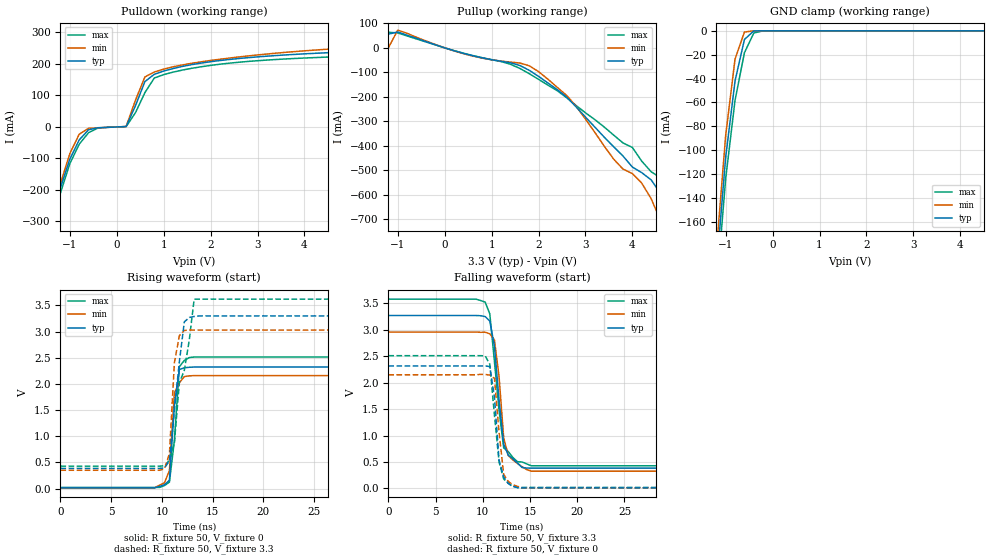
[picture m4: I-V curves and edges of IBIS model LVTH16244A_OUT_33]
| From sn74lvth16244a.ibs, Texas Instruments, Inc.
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|  Model LVTH16244A OUTPUT_33
[Model]   LVTH16244A_OUT_33
Model_type  3-state
Polarity   Inverting
Enable   Active-Low
Vmeas = 1.5V
Cref = 50pF
Rref = 500
Vref = 0
| variable   typ   min   max
C_comp   9pf   NA   NA
[Temperature Range]   40   -25   100
| Ambient temperature   25   -40   85
[Voltage range]   3.3   3.0   3.6
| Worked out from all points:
|   slope of the pulldown table from 0 to 0.495 V, typ, clamps not added: 4.75 ohm
|   slope of the pullup table from 0 to 0.495 V, typ, clamps not added: 18.1 ohm
|   GND clamp passes 1 mA (typ) near -0.43 V on its own axis
|   rising waveform, R_fixture 50, V_fixture 0: 20-80 % time 578ps typ, 424ps min, 626ps max; typ from 0.013 V to 2.32 V
|   falling waveform, R_fixture 50, V_fixture 3.3: 20-80 % time 906ps typ, 867ps min, 1.08ns max; typ from 3.27 V to 0.384 V
|   rising waveform, R_fixture 50, V_fixture 3.3: 20-80 % time 946ps typ, 513ps min, 1.47ns max; typ from 0.386 V to 3.3 V
|   falling waveform, R_fixture 50, V_fixture 0: 20-80 % time 696ps typ, 699ps min, 798ps max; typ from 2.32 V to 0.01 V
[Pullup]
|  Voltage   I(typ)   I(min)   I(max)
-5V       75.18uA    69.08uA    78.73uA
-2V       66.13uA    58.35uA    71.21uA
-1.8V     54.42mA    58.13uA    70.93uA
-1.6V     54.34mA    57.93uA    70.68uA
-1.2V     55.85mA    57.48uA    63.46mA
-1V       64.85mA    72.21mA    61.01mA
2V        -116.5mA   -96.95mA   -128.6mA
4.2V      -509.9mA   -552.6mA   -463mA
4.6V      -594.6mA   -704.6mA   -530.6mA
5V        -741.4mA   -898.7mA   -629.6mA
5.4V      -902.7mA   -1.093A    -764.1mA
10V       -2.757A    -3.325A    -2.409A
[Pulldown]
|   Voltage   I(typ)   I(min)   I(max)
-5V       -2.912A    -3.255A    -2.64A
-1.4V     -305mA     -304mA     -322.6mA
-1V       -102.1mA   -84.75mA   -116.6mA
-800mV    -41.16mA   -23.1mA    -54.85mA
-400mV    -2.567mA   -2.87mA    -3.477mA
200mV     1.27mA     1.375mA    1.238mA
600mV     144.1mA    158.7mA    109.1mA
800mV     167mA      174.3mA    155.3mA
1V        177.4mA    183.6mA    166.1mA
2.8V      220mA      225.5mA    208mA
8V        280.7mA    314.1mA    253.6mA
10V       322.3mA    360.9mA    281.2mA
[GND Clamp]
|   Voltage   I(typ)   I(min)   I(max)
-5V       -2.807A    -3.113A    -2.569A
-1.2V     -200.9mA   -185.7mA   -219.7mA
-1V       -106mA     -87.66mA   -123.8mA
-800mV    -41.92mA   -23.57mA   -58.05mA
-600mV    -7.219mA   -1.025mA   -18.33mA
-400mV    -92.45uA   -1.314uA   -1.828mA
-200mV    -117.2nA   -1.107nA   -13.84uA
5V        500.4pA    11.26nA    49.47nA
[ramp]
| variable   typ   min   max
dV/dt_r   1.470E+00/5.510E-10  1.338E+00/5.700E-10  1.608E+00/4.880E-10
dV/dt_f   1.764E+00/5.300E-10  1.584E+00/4.880E-10  1.922E+00/5.410E-10
R_load = 50
[Rising Waveform]
R_fixture = 50
V_fixture = 0
V_fixture_min = 0
V_fixture_max = 0
C_fixture = 0
L_fixture = 0
|   Time   V(typ)   V(min)   V(max)
0s        12.64mV    12.94mV    20.38mV
9.277ns   12.64mV    12.94mV    20.38mV
9.766ns   41.76mV    65.18mV    21.73mV
10.25ns   71.66mV    108mV      55.58mV
10.74ns   158.2mV    344.5mV    122.8mV
11.23ns   1.583V     1.834V     917.5mV
11.72ns   2.276V     2.021V     2.33V
12.21ns   2.309V     2.14V      2.449V
12.7ns    2.318V     2.154V     2.504V
49.71ns   2.323V     2.159V     2.514V
[Falling Waveform]
R_fixture = 50
V_fixture = 3.3
V_fixture_min = 3
V_fixture_max = 3.6
C_fixture = 0pf
L_fixture = 0nH
|   Time   V(typ)   V(min)   V(max)
0s        3.272V     2.959V     3.582V
10.25ns   3.252V     2.956V     3.525V
10.74ns   3.166V     2.925V     3.303V
11.23ns   2.696V     2.808V     2.403V
11.72ns   1.674V     2.115V     1.478V
12.21ns   837.1mV    957.4mV    766.5mV
12.7ns    627.9mV    620.3mV    696.3mV
13.67ns   480.2mV    470.7mV    504.9mV
15.14ns   383.6mV    325.6mV    428.1mV
49.71ns   383.6mV    325.6mV    428.1mV
[Rising Waveform]
R_fixture = 50
V_fixture = 3.3
V_fixture_min = 3
V_fixture_max = 3.6
C_fixture = 0pf
L_fixture = 0nH
|   Time   V(typ)   V(min)   V(max)
0s        386.3mV    349.2mV    427.7mV
9.766ns   386.3mV    349.2mV    427.7mV
10.25ns   391.8mV    375.5mV    434.8mV
10.74ns   529.8mV    662.7mV    539.9mV
11.23ns   1.498V     2.403V     877.9mV
11.72ns   2.425V     2.924V     2.027V
12.21ns   3.186V     3.022V     2.259V
12.7ns    3.27V      3.03V      2.845V
13.18ns   3.289V     3.03V      3.621V
49.71ns   3.3V       3.03V      3.621V
[Falling Waveform]
R_fixture = 50
V_fixture = 0
V_fixture_min = 0
V_fixture_max = 0
C_fixture = 0pf
L_fixture = 0nH
|   Time   V(typ)   V(min)   V(max)
0s        2.317V     2.15V      2.512V
10.25ns   2.318V     2.156V     2.507V
10.74ns   2.306V     2.145V     2.351V
11.23ns   1.726V     2.086V     1.389V
11.72ns   534.5mV    1.062V     500mV
12.21ns   214.7mV    265.5mV    178.6mV
12.7ns    93.09mV    128.8mV    95.22mV
13.18ns   45.46mV    69.1mV     31.28mV
14.16ns   10.14mV    12.09mV    18.79mV
49.71ns   10.14mV    12.09mV    18.79mV
